(* Logix 5000 AddOnInstructionDefinition export YAI_Assy_72_73_118_EIP_Hz; software revision 21.03 *)

ADD_ON_INSTRUCTION YAI_Assy_72_73_118_EIP_Hz   (* revision 1.0, vendor Yaskawa America, Inc. *)
// YAI Assembly 72/73 and 118
// Help:
// This add-on instruction is for use with input assemblie 72/73 and output assemblies 118.
// Node_Input_Assy is defined as the node's input assembly integer array.
// Node_Output_Assy is defined as the node's output assembly integer array.
// Torque limit/reference, torque compensation and torque output variables are only available with A1000.
VAR_IN_OUT
   Node_Input_Assy : AB:ETHERNET_MODULE_INT_6Bytes:I:0; {required}   // Input assembly words
   Node_Output_Assy : AB:ETHERNET_MODULE_INT_12Bytes:O:0; {required}   // Output assembly words
END_VAR
VAR_INPUT
   RunFwd : BOOL; {visible}   // Forward run command
   RunRev : BOOL; {visible}   // Reverse run command
   MFI_3 : BOOL; {visible}   // Multi-function input 3
   MFI_4 : BOOL; {visible}   // Multi-function input 4
   MFI_5 : BOOL; {visible}   // Multi-function input 5
   MFI_6 : BOOL; {visible}   // Multi-function input 6
   MFI_7 : BOOL; {visible}   // Multi-function input 7
   MFI_8 : BOOL; {visible}   // Multi-function input 8
   External_Fault : BOOL;   // External fault command (EF0)
   FaultReset : BOOL; {visible}   // Fault reset command
   MFO_1 : BOOL; {visible}   // Multi-function output (M1-M2 for A/P1000, MA/MB/MC for V1000)
   MFO_2 : BOOL; {visible}   // Multi-function output (M3-M4 for A/P1000, P1 for V1000)
   MFO_3 : BOOL; {visible}   // Multi-function output (M5-M6 for A/P1000, P2 for V1000)
   Freq_Ref : REAL; {visible}   // Frequency reference command in Hz (xx.xx resolution)
   Digital_Output_Fault_Enable : BOOL;   // Bit to enable control of fault output relay over the network
   Custom_Out_1 : INT;
   Custom_Out_2 : INT;
   Custom_Out_3 : INT;
   Custom_Out_4 : INT;
END_VAR
VAR_OUTPUT
   Faulted : BOOL; {access Read Only, visible}   // Drive faulted status bit
   Output_Freq : REAL; {access Read Only, visible}   // Drive output frequency in Hz (xx.xx resolution)
   RunningFwd : BOOL; {access Read Only, visible}   // Drive running forward status bit
   Faulted1 : BOOL; {access Read Only, visible}   // Drive faulted status bit
   NetCtrlStatus : BOOL; {access Read Only, visible}   // Drive network run source status bit (1 = source coming from network)
   NetRefStatus : BOOL; {access Read Only, visible}   // Drive network reference status bit (1 = reference coming from network)
   Output_Freq1 : REAL; {access Read Only, visible}   // Drive output frequency in Hz (xx.xx resolution)
   Ready : BOOL; {access Read Only, visible}   // Drive ready status bit
   RunningFwd1 : BOOL; {access Read Only, visible}   // Drive running forward status bit
   RunningRev : BOOL; {access Read Only, visible}   // Drive running reverse status bit
   Torque_Actual : REAL; {access Read Only, visible}   // Drive torque output in engineering units.
   Warning : BOOL; {access Read Only, visible}   // Drive warning (alarm) status bit
   At_Speed : BOOL; {access Read Only, visible}   // Drive at commanded speed status bit
   Drive_State : INT; {access Read Only}   // Drive Status - Refer to class 0x29, Instance 0x1, Attribute 0x6 for details
END_VAR
VAR_INPUT
   Motor_Rated_Torq : REAL := 100.0; {visible}   // Motor rated torque (Engineering units)
END_VAR
VAR
   FRef_Convert : DINT;
   FOut_Convert : REAL;
   FOut_Temp : REAL;
   TRef_Convert : INT;
   TComp_Convert : INT;
   TOut_Convert : REAL;
   TOut_Temp : REAL;
   IOut_Temp : REAL;
   IOut_Convert : REAL;
   AO1_Convert : INT;
   AO2_Convert : INT;
   Motor_Speed_Temp : REAL;
   Motor_Speed_Convert : REAL;
   Freq_Cmd_Temp : REAL;
   Freq_Cmd_Convert : REAL;
   AI1_Temp : REAL;
   AI1_Convert : REAL;
   AI2_Temp : REAL; {access None}
   AI2_Convert : REAL; {access None}
   AI3_Temp : REAL; {access None}
   AI3_Convert : REAL; {access None}
   DriveStatusTempBits : INT;
   Tout_Convert_Temp : REAL;
END_VAR

ROUTINE Logic   (* ladder *)
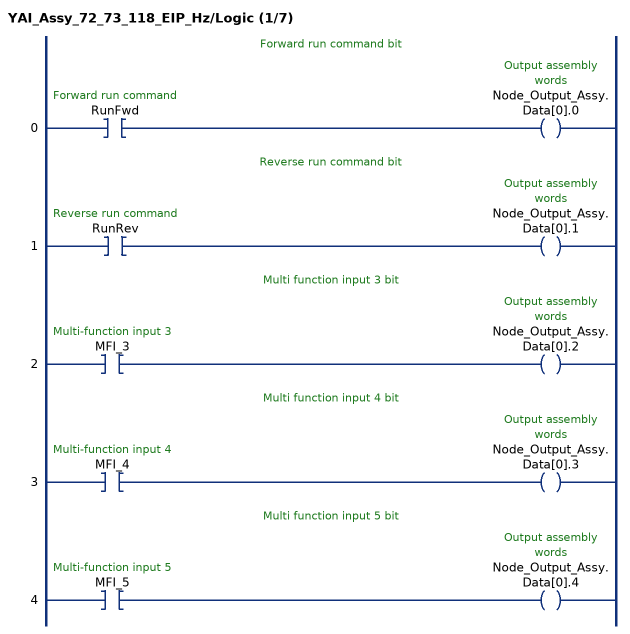
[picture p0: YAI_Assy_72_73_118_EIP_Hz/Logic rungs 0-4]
   // Forward run command bit
   0: XIC(RunFwd)OTE(Node_Output_Assy.Data[0].0);
   // Reverse run command bit
   1: XIC(RunRev)OTE(Node_Output_Assy.Data[0].1);
   // Multi function input 3 bit
   2: XIC(MFI_3)OTE(Node_Output_Assy.Data[0].2);
   // Multi function input 4 bit
   3: XIC(MFI_4)OTE(Node_Output_Assy.Data[0].3);
   // Multi function input 5 bit
   4: XIC(MFI_5)OTE(Node_Output_Assy.Data[0].4);
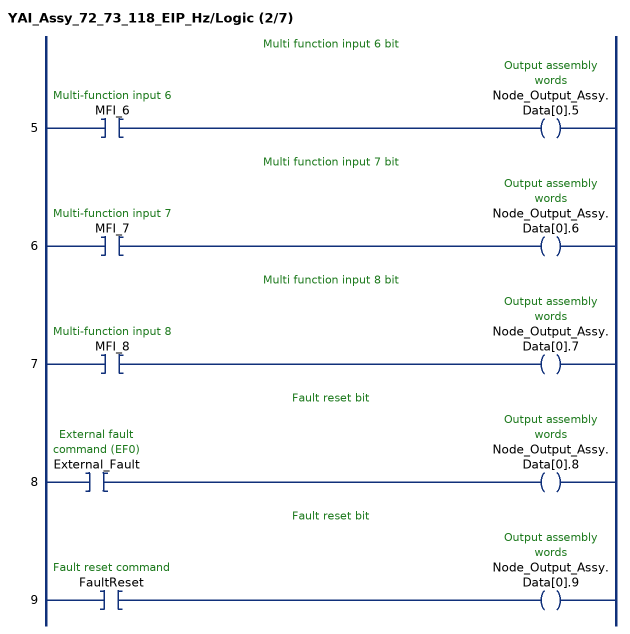
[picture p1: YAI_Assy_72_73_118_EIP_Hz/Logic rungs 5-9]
   // Multi function input 6 bit
   5: XIC(MFI_6)OTE(Node_Output_Assy.Data[0].5);
   // Multi function input 7 bit
   6: XIC(MFI_7)OTE(Node_Output_Assy.Data[0].6);
   // Multi function input 8 bit
   7: XIC(MFI_8)OTE(Node_Output_Assy.Data[0].7);
   // Fault reset bit
   8: XIC(External_Fault)OTE(Node_Output_Assy.Data[0].8);
   // Fault reset bit
   9: XIC(FaultReset)OTE(Node_Output_Assy.Data[0].9);
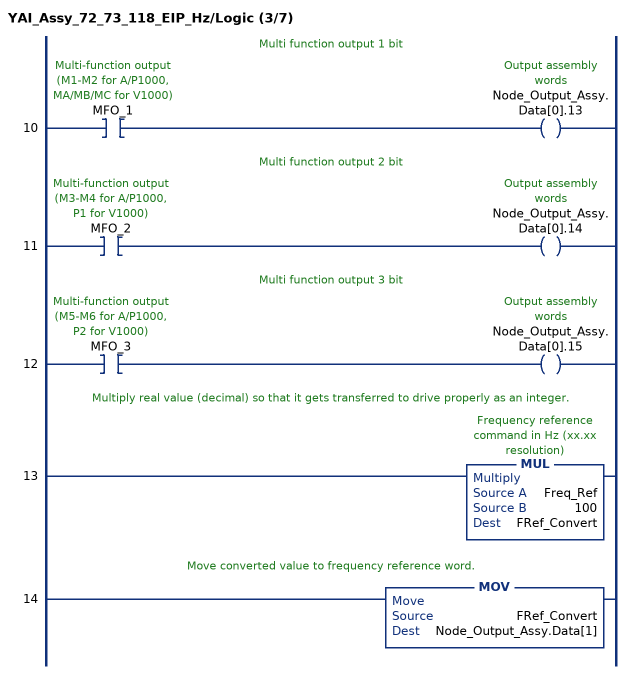
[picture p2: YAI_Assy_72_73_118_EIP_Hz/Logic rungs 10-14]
   // Multi function output 1 bit
   10: XIC(MFO_1)OTE(Node_Output_Assy.Data[0].13);
   // Multi function output 2 bit
   11: XIC(MFO_2)OTE(Node_Output_Assy.Data[0].14);
   // Multi function output 3 bit
   12: XIC(MFO_3)OTE(Node_Output_Assy.Data[0].15);
   // Multiply real value (decimal) so that it gets transferred to drive properly as an integer.
   13: MUL(Freq_Ref,100,FRef_Convert);
   // Move converted value to frequency reference word.
   14: MOV(FRef_Convert,Node_Output_Assy.Data[1]);
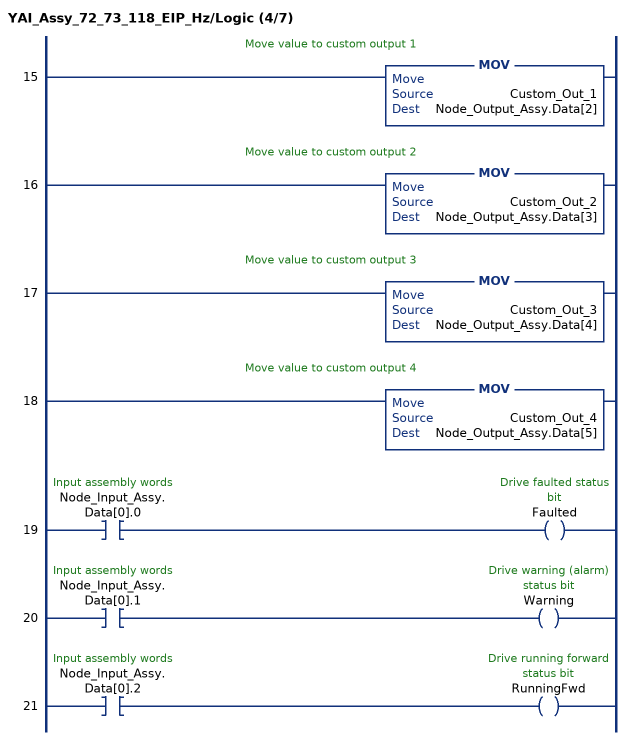
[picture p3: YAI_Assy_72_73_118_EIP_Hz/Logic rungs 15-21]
   // Move value to custom output 1
   15: MOV(Custom_Out_1,Node_Output_Assy.Data[2]);
   // Move value to custom output 2
   16: MOV(Custom_Out_2,Node_Output_Assy.Data[3]);
   // Move value to custom output 3
   17: MOV(Custom_Out_3,Node_Output_Assy.Data[4]);
   // Move value to custom output 4
   18: MOV(Custom_Out_4,Node_Output_Assy.Data[5]);
   19: XIC(Node_Input_Assy.Data[0].0)OTE(Faulted);
   20: XIC(Node_Input_Assy.Data[0].1)OTE(Warning);
   21: XIC(Node_Input_Assy.Data[0].2)OTE(RunningFwd);
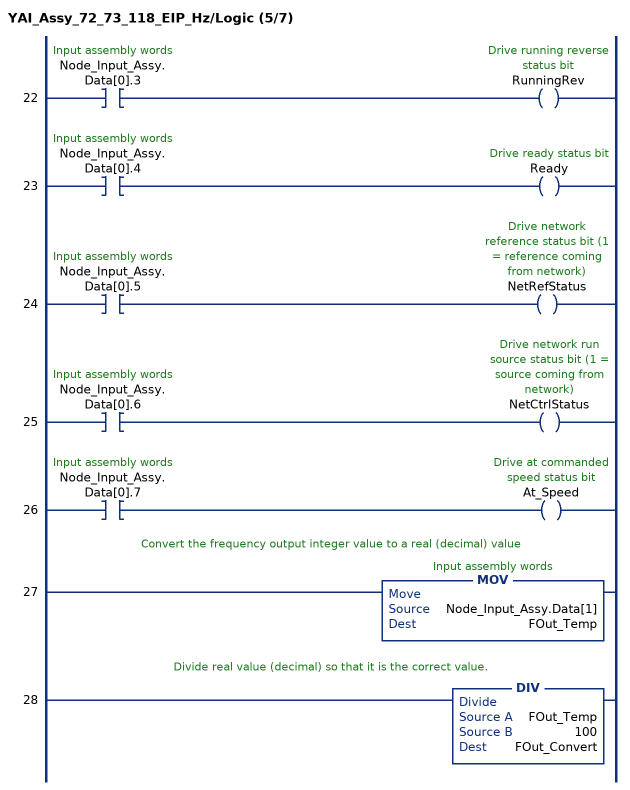
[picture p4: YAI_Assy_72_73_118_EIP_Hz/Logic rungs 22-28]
   22: XIC(Node_Input_Assy.Data[0].3)OTE(RunningRev);
   23: XIC(Node_Input_Assy.Data[0].4)OTE(Ready);
   24: XIC(Node_Input_Assy.Data[0].5)OTE(NetRefStatus);
   25: XIC(Node_Input_Assy.Data[0].6)OTE(NetCtrlStatus);
   26: XIC(Node_Input_Assy.Data[0].7)OTE(At_Speed);
   // Convert the frequency output integer value to a real (decimal) value
   27: MOV(Node_Input_Assy.Data[1],FOut_Temp);
   // Divide real value (decimal) so that it is the correct value.
   28: DIV(FOut_Temp,100,FOut_Convert);
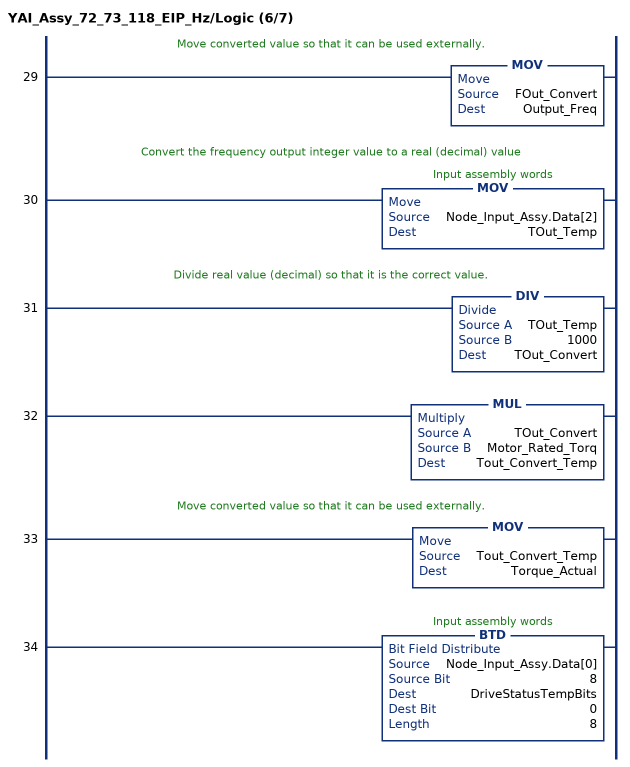
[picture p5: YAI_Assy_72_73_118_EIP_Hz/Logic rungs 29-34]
   // Move converted value so that it can be used externally.
   29: MOV(FOut_Convert,Output_Freq);
   // Convert the frequency output integer value to a real (decimal) value
   30: MOV(Node_Input_Assy.Data[2],TOut_Temp);
   // Divide real value (decimal) so that it is the correct value.
   31: DIV(TOut_Temp,1000,TOut_Convert);
   32: MUL(TOut_Convert,Motor_Rated_Torq,Tout_Convert_Temp);
   // Move converted value so that it can be used externally.
   33: MOV(Tout_Convert_Temp,Torque_Actual);
   34: BTD(Node_Input_Assy.Data[0],8,DriveStatusTempBits,0,8);
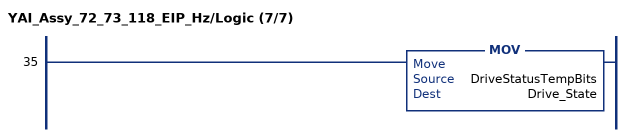
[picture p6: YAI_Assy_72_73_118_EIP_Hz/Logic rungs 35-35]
   35: MOV(DriveStatusTempBits,Drive_State);
END_ROUTINE
END_ADD_ON_INSTRUCTION
